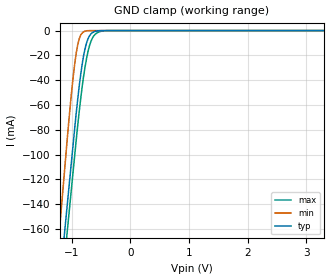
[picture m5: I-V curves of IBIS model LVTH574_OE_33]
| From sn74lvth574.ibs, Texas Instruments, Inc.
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[Model]   LVTH574_OE_33
Model_type  Input
Vinl = 0.8
Vinh = 2.34
| variable   typ   min   max
C_comp   4.05pF   3.22pF   5.48pF
[Temperature Range]   40   -40   100
| Ambient temperature   25   -40   85
[Voltage range]   3.3   3   3.6
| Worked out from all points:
|   GND clamp passes 1 mA (typ) near -0.62 V on its own axis
[GND Clamp]
| LVTH574_OE_33
|   Voltage   I(typ)   I(min)   I(max)
-5.5V     -2.407A    -2.649A    -2.406A
-1.22V    -209.3mA   -166mA     -230mA
-1.205V   -202mA     -157.6mA   -222.8mA
-1.125V   -163.1mA   -113mA     -184.2mA
-1.075V   -138.8mA   -85.25mA   -160.1mA
-975mV    -90.17mA   -36.12mA   -112mA
-900mV    -55.28mA   -11.44mA   -76.47mA
-825mV    -27.42mA   -1.98mA    -45.67mA
-775mV    -14.64mA   -464.8uA   -29.41mA
-650mV    -1.684mA   -2.076uA   -6.132mA
-395mV    -1.224uA   -43.32pA   -35.77uA
3.3V      16.15pA    8.657pA    1.272nA
